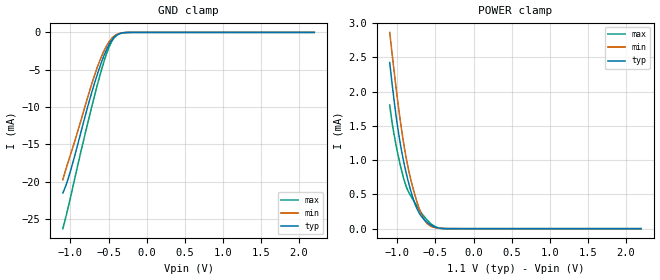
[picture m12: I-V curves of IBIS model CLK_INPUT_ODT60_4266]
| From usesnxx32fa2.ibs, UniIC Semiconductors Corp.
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| CLK_INPUT_ODT60_4266 (with 60ohm ODT, 3200-4266Mbps)
[Model]   CLK_INPUT_ODT60_4266
Model_type   Input
Vinl = 110.833mV
Vinh = 255.833mV
|   typ   min   max
|C_comp   0.641pF   0.591pF   0.704pF
C_comp_power_clamp   0.3205pF   0.2955pF   0.3520pF
C_comp_gnd_clamp   0.3205pF   0.2955pF   0.3520pF
| Note: C_comp changes when the ODT circuit is enabled.
[Model Spec]
| Input threshold voltage corners
Vinl   0.1108V   0.1042V   0.1225V
Vinh   0.2558V   0.2492V   0.2675V
| Dynamic Overshoot Parameters from LPDDR4 Specification
D_overshoot_ampl_h   0.30   NA   NA
D_overshoot_ampl_l   0.30   NA   NA
D_overshoot_area_h   0.1n   NA   NA
D_overshoot_area_l   0.1n   NA   NA
[Voltage Range]   1.1000V   1.0600V   1.1700V
[POWER Clamp Reference]   1.1000V   1.0600V   1.1700V
| Junction Temperature (Ambient temp is 35C typ 95C min -40C max)
[Temperature Range]   50.0   110.0   -40.0
[Add Submodel]
| Submodel Name   Mode
60ohm_ODT_4266   Non-Driving
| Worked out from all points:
|   GND clamp passes 1 mA (typ) near -0.45 V on its own axis
|   POWER clamp passes 1 mA (typ) near -0.92 V on its own axis
[GND Clamp]
|   Voltage   I(typ)   I(min)   I(max)
-1.1V     -21.49mA   -19.74mA   -26.28mA
-1.05V    -20.21mA   -18mA      -24.3mA
-1.001V   -18.6mA    -16.41mA   -22.15mA
-760.1mV  -9.441mA   -8.207mA   -11.59mA
-690.8mV  -7.023mA   -5.938mA   -8.749mA
-611.6mV  -4.528mA   -3.695mA   -5.689mA
-558.8mV  -3.072mA   -2.454mA   -3.854mA
-492.8mV  -1.616mA   -1.25mA    -1.96mA
-449.9mV  -937.2uA   -717.2uA   -1.077mA
-393.8mV  -384.3uA   -286.1uA   -384.4uA
-218.9mV  -5.073uA   -4.963uA   -2.555uA
2.2V      0A         0A         0A
[POWER Clamp]
|   Voltage   I(typ)   I(min)   I(max)
-1.1V     2.422mA    2.862mA    1.802mA
-1.064V   2.064mA    2.5mA      1.513mA
-991.1mV  1.446mA    1.826mA    1.078mA
-935mV    1.079mA    1.372mA    807.4uA
-872.3mV  757.9uA    964uA      583.2uA
-786.5mV  417uA      559.2uA    407.8uA
-723.8mV  249.1uA    325.9uA    295uA
-667.7mV  157.6uA    169.9uA    204.9uA
-591.8mV  77.95uA    60.06uA    105.2uA
-492.8mV  18.73uA    10.94uA    23.72uA
-383.9mV  1.579uA    1.072uA    1.286uA
2.2V      0A         0A         0A
